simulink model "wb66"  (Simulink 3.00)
settings: Solver=ode45  SolverMode=SingleTasking  StartTime=0.0  StopTime=30  RelTol=1e-3  AbsTol=1e-6

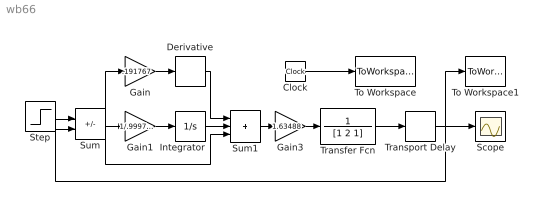
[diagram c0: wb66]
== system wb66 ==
  Clock : Clock
  Derivative : Derivative
  Gain : Gain  Gain=.191767  SaturateOnIntegerOverflow=on
  Gain1 : Gain  Gain=1/.9997325  SaturateOnIntegerOverflow=on
  Gain3 : Gain  Gain=1.63488  SaturateOnIntegerOverflow=on
  Integrator : Integrator  ExternalReset=none  InitialConditionSource=internal  InitialCondition=0  LimitOutput=off  UpperSaturationLimit=inf  LowerSaturationLimit=-inf  ShowSaturationPort=off  ShowStatePort=off  AbsoluteTolerance=auto
  Scope : Scope
  Step : Step  Time=0  Before=0  After=1  SampleTime=0
  Sum : Sum  Inputs=+-  SaturateOnIntegerOverflow=on
  Sum1 : Sum  Inputs=+++  SaturateOnIntegerOverflow=on
  To Workspace : ToWorkspace  VariableName=t  SampleTime=-1  SaveFormat=Matrix
  To Workspace1 : ToWorkspace  VariableName=y  SampleTime=-1  SaveFormat=Matrix
  Transfer Fcn : TransferFcn  Numerator=1  Denominator=[1 2 1]
  Transport Delay : TransportDelay  DelayTime=.5  InitialInput=0  BufferSize=1024
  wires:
  Derivative/1 -> Sum1/1
  Integrator/1 -> Sum1/2
  Gain1/1 -> Integrator/1
  Gain/1 -> Derivative/1
  Sum/1 -> Sum1/3, Gain1/1, Gain/1
  Step/1 -> Sum/1
  Clock/1 -> To Workspace/1
  Transfer Fcn/1 -> Transport Delay/1
  Transport Delay/1 -> Scope/1, To Workspace1/1, Sum/2
  Sum1/1 -> Gain3/1
  Gain3/1 -> Transfer Fcn/1
